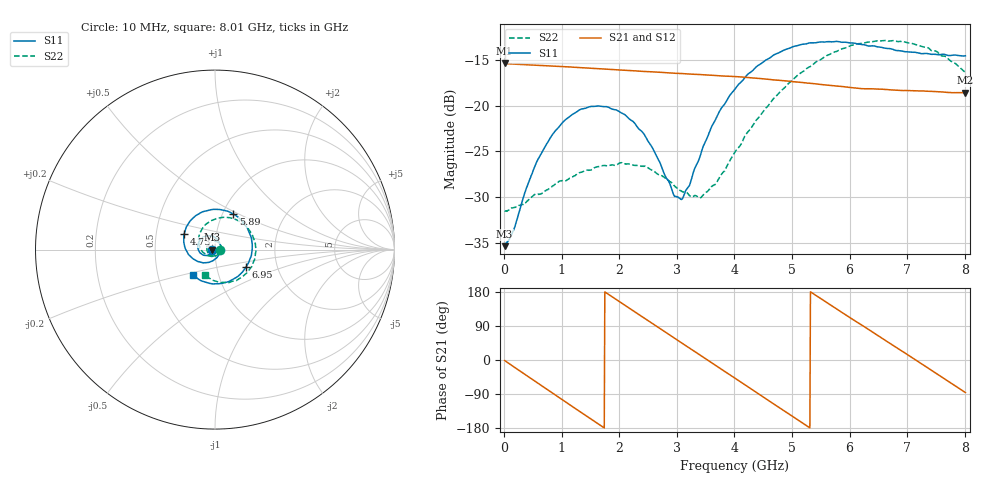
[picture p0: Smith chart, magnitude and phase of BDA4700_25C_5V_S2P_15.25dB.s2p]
!Agilent Technologies,E5071B,MY42404982,A.09.10
!Date: Mon Oct 20 13:33:51 2025
!Data & Calibration Information:
!Freq	S11:SOLT2(ON)	S21:SOLT2(ON)	S12:SOLT2(ON)	S22:SOLT2(ON)
# Hz S RI R 50
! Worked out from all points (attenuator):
!   801 points, 10 MHz to 8.01 GHz, reference 50 ohm
!   highest |S21| = -15.35 dB at 10 MHz (marker M1); lowest = -18.6 dB at 8 GHz (marker M2)
!   lowest |S11| = -35.4 dB at 10 MHz (marker M3), VSWR 1.03, Z = 48.3 - j0.107 ohm
!   |S11| at or under -10 dB: start of sweep to end of sweep
!   |S22| runs from -31.6 to -12.8 dB; largest |S21 - S12| = 0.0013
!   S11 on the Smith chart (normalised r, x): 10 MHz: 0.97, -0.00; 4.73 GHz: 0.70, +0.13; 5.89 GHz: 1.12, +0.47; 6.95 GHz: 1.38, -0.28; 8.01 GHz: 0.75, -0.22
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1e7  -0.017 -0.00111  0.1707 -0.00369  0.1707 -0.00388  0.0265 -0.00104
1.6e8  -0.018 -0.00998  0.162 -0.0495  0.1619 -0.0496  0.0264 -0.00797
4.2e8  -0.0278 -0.0253  0.1207 -0.1166  0.1207 -0.1166  0.0196 -0.0232
7e8  -0.0486 -0.0329  0.0489 -0.1587  0.0489 -0.1588  0.00417 -0.0337
1.03e9  -0.0787 -0.0223  -0.0472 -0.157  -0.0473 -0.157  -0.0205 -0.0329
1.35e9  -0.0958 0.00723  -0.123 -0.1051  -0.1232 -0.1052  -0.0408 -0.0143
2.09e9  -0.0477 0.0759  -0.1286 0.0895  -0.1288 0.0896  -0.0233 0.0421
2.42e9  -0.00462 0.0707  -0.0574 0.1434  -0.0574 0.1434  0.00615 0.0461
2.68e9  0.0213 0.0459  0.0116 0.1523  0.0115 0.1524  0.0247 0.0339
2.95e9  0.0311 0.00837  0.0789 0.1287  0.0789 0.1286  0.0339 0.0137
3.09e9  0.0282 -0.0122  0.1074 0.1051  0.107 0.1054  0.0339 0.000451
3.43e9  -0.00377 -0.0562  0.1459 0.0265  0.146 0.0265  0.0167 -0.0269
3.75e9  -0.0588 -0.0737  0.1355 -0.0542  0.1356 -0.0544  -0.0154 -0.0381
4.01e9  -0.1082 -0.0598  0.0966 -0.1076  0.0966 -0.1075  -0.0461 -0.0311
4.73e9  -0.1724 0.087  -0.0708 -0.1188  -0.0706 -0.1192  -0.0903 0.0689
5.35e9  -0.0616 0.2127  -0.1323 0.00716  -0.1324 0.00672  -0.00699 0.1665
5.89e9  0.1011 0.199  -0.0699 0.1065  -0.07 0.1064  0.128 0.1618
6.68e9  0.2051 -0.0183  0.0853 0.0879  0.0856 0.0879  0.2252 -0.0256
6.95e9  0.172 -0.0989  0.1143 0.0407  0.1145 0.0401  0.2015 -0.0988
7.48e9  0.0299 -0.1892  0.1002 -0.0654  0.1004 -0.0657  0.0782 -0.1838
8e9  -0.1225 -0.1426  0.0105 -0.1174  0.0107 -0.1176  -0.0508 -0.1444
8.01e9  -0.1247 -0.1407  0.00854 -0.1176  0.00864 -0.1177  -0.053 -0.1425
